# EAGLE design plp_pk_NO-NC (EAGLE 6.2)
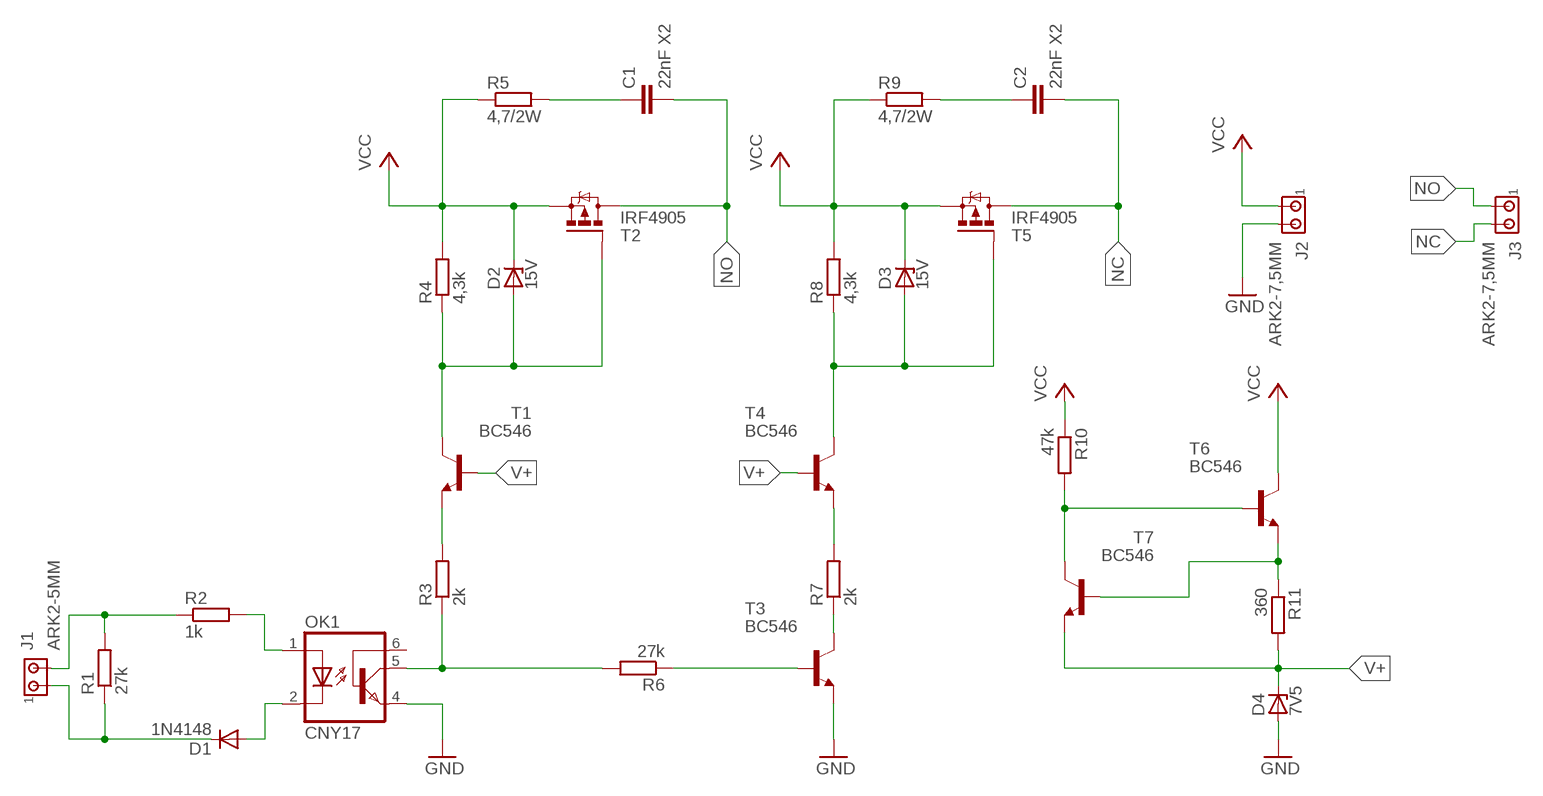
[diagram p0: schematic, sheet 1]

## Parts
C1  22nF X2  C-EU102-054X133  [C102-054X133]
C2  22nF X2  C-EU102-054X133  [C102-054X133]
D1  1N4148  1N4148DO35-7  [DO35-7]
D2  15V  ZENER-DIODEDO34-7  [DO34Z7]
D3  15V  ZENER-DIODEDO34-7  [DO34Z7]
D4  7V5  ZENER-DIODEDO34-7  [DO34Z7]
J1  ARK2-5MM  [2PIN-5MM]
J2  ARK2-7,5MM  [2PIN-7,5MM]
J3  ARK2-7,5MM  [2PIN-7,5MM]
OK1  CNY17  [DIL06]
R1  27k  R-EU_0207/7  [0207/7]
R2  1k  R-EU_0207/7  [0207/7]
R3  2k  R-EU_0207/7  [0207/7]
R4  4,3k  R-EU_0207/7  [0207/7]
R5  4,7/2W  R-EU_0613/5V  [P0613V]
R6  27k  R-EU_0207/7  [0207/7]
R7  2k  R-EU_0207/7  [0207/7]
R8  4,3k  R-EU_0207/7  [0207/7]
R9  4,7/2W  R-EU_0613/5V  [P0613V]
R10  47k  R-EU_0207/7  [0207/7]
R11  360  R-EU_0207/7  [0207/7]
T1  BC546  MPSA42-NPN-TO92-CBE  [TO92-CBE]
T2  IRF4905  IRF9530  [TO220BV]
T3  BC546  MPSA42-NPN-TO92-CBE  [TO92-CBE]
T4  BC546  MPSA42-NPN-TO92-CBE  [TO92-CBE]
T5  IRF4905  IRF9530  [TO220BV]
T6  BC546  MPSA42-NPN-TO92-CBE  [TO92-CBE]
T7  BC546  MPSA42-NPN-TO92-CBE  [TO92-CBE]

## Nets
GND: D4.A J2.P2 OK1.4(EMI) T3.E
N$1: OK1.1(A) R2.2
N$2: D1.A OK1.2(C)
N$3: D1.C J1.P$1 R1.1
N$4: J1.P$2 R1.2 R2.1
N$5: OK1.5(COL) R3.1 R6.2
N$6: R3.2 T1.E
N$7: D2.A R4.1 T1.C T2.G
N$8: C1.1 R5.2
N$9: R11.1 T6.E T7.B
N$10: R6.1 T3.B
N$11: R7.1 T3.C
N$12: D3.A R8.1 T4.C T5.G
N$13: R7.2 T4.E
N$14: C2.1 R9.2
N$18: R10.2 T6.B T7.C
NC: C2.2 J3.P2 T5.D
NO: C1.2 J3.P1 T2.D
V+: D4.C R11.2 T1.B T4.B T7.E
VCC: D2.C D3.C J2.P1 R4.2 R5.1 R8.2 R9.1 R10.1 T2.S T5.S T6.C
Unconnected: OK1.6(BAS)

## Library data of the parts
C1 C2 = rcl:C-EU: CAPACITOR, European symbol
D1 = diode:1N4148: DIODE
D2-D4 = diode:ZENER-DIODE: Z-Diode
J1-J3 = zlacza_futrzak:ARK2: ARK 2
OK1 = optocoupler:CNY17: SIEMENS OPTO COUPLER; MPN: CNY17-1; OC_FARNELL: 1045399; OC_NEWARK: 05M4044
R1-R11 = rcl:R-EU_: RESISTOR, European symbol
T1 T3 T4 T6 T7 = transistor:*-NPN-: NPN Transistror BF959 corrected 2008.03.06
T2 T5 = transistor-power:IRF9530: P-CHANNEL HEXFET POWER-MOS-FET Source: http://www.irf.com/product-info/datasheets/data/irf9530.pdf

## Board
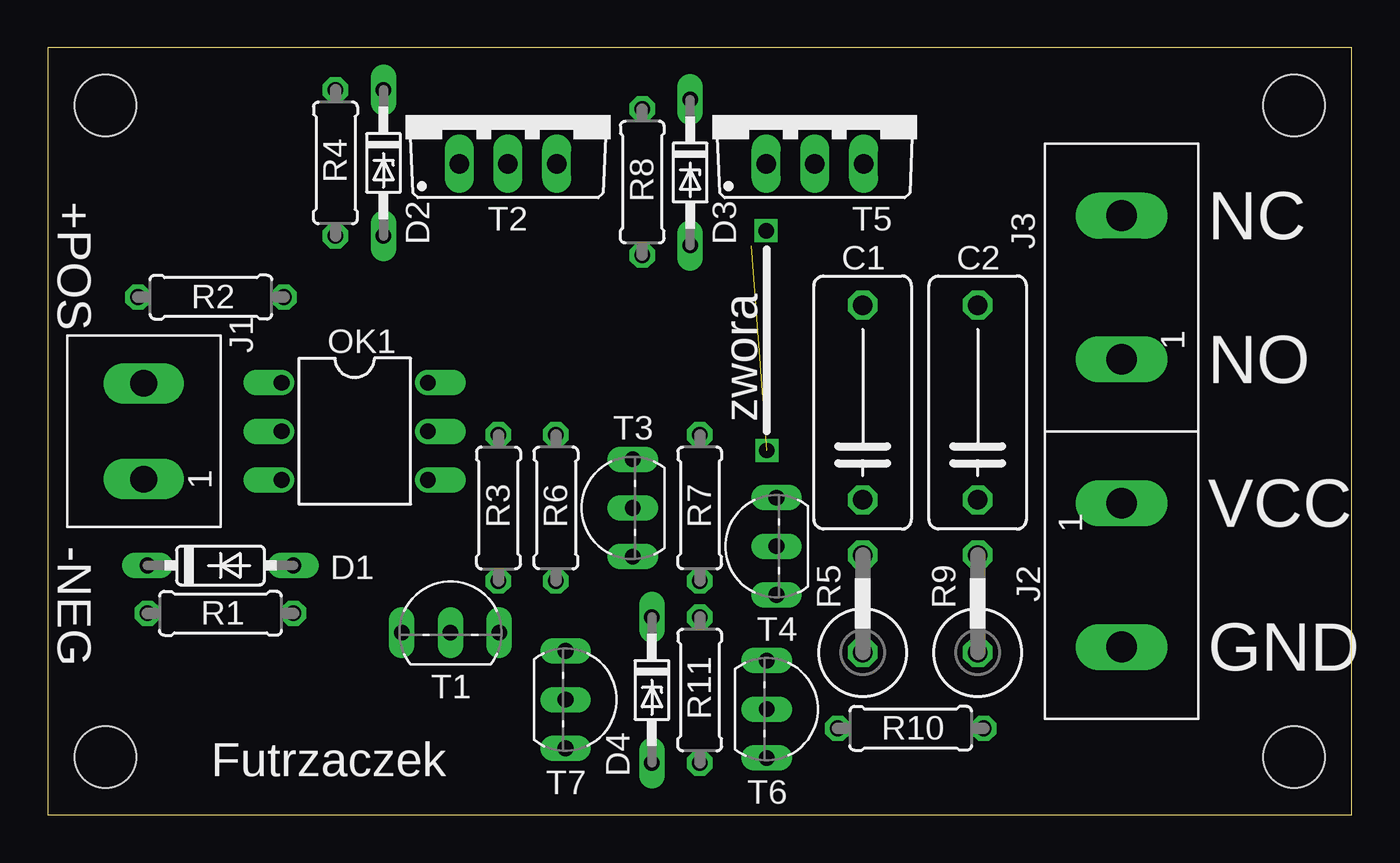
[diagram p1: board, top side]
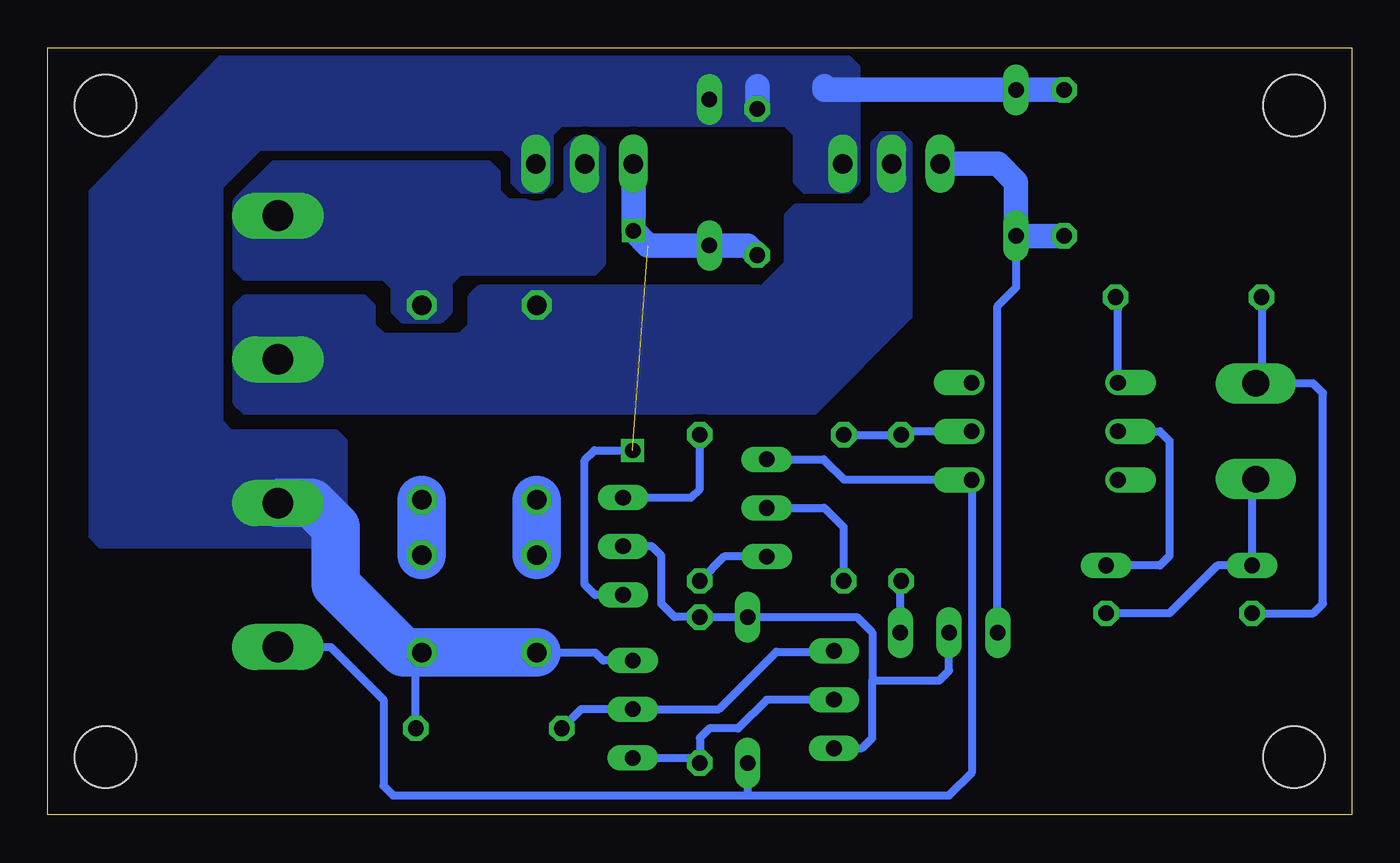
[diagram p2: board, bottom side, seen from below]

Size 68 x 40 mm. Coordinates in mm from the lower left corner, seen from the top.
Outline: 0,0 68,0 68,40 0,40 0,0
Copper layers (1*16): Top 0.035mm / dielectric 1.5mm / Bottom 0.035mm
Design rules: minimum track width 10mil, minimum drill 24mil, track to track 8mil, track to pad 8mil, pad to pad 8mil, via to via 8mil, smd to smd 8mil, copper to edge 10mil, drill to drill 8mil, minimum pad ring 10mil, minimum via ring 8mil, stop-mask expansion 4mil, vias tented up to drill 0mil, thermal gap 10mil
Holes 3.2 mm at 3,3 3,37 65,37 65,3

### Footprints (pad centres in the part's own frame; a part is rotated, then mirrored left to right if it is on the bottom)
C102-054X133 = drill 1.016 octagon: 1 -5.08,0; 2 5.08,0
DO35-7 = drill 0.813 long: A 3.81,0; C -3.81,0
DO34Z7 = drill 0.813 long: A 3.81,0; C -3.81,0
2PIN-5MM = drill 1.4 long: P$1 -2.5,0; P$2 2.5,0
2PIN-7,5MM = drill 1.6 long: P1 -3.75,0; P2 3.75,0
DIL06 = drill 0.813 offset: 1 -2.54,-3.81; 2 0,-3.81; 3 2.54,-3.81; 4 2.54,3.81; 5 0,3.81; 6 -2.54,3.81
0207/7 = drill 0.813 octagon: 1 -3.81,0; 2 3.81,0
P0613V = drill 1.016 octagon: 1 -2.54,0; 2 2.54,0
TO92-CBE = drill 0.813 long: B 0,0; C -2.54,0; E 2.54,0
TO220BV = drill 1.016 long: D 0,-2.54; G -2.54,-2.54; S 2.54,-2.54

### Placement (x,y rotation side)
C1  42.5,21.5 90 top
C2  48.5,21.5 90 top
D1  9,13 0 top
D2  17.5,34 270 top
D3  33.5,33.5 270 top
D4  31.5,6.5 270 top
J1  5,20 90 top
J2  56,12.5 270 top
J3  56,27.5 90 top
OK1  16,20 270 top
R1  9,10.5 180 top
R2  8.5,27 0 top
R3  23.5,16 270 top
R4  15,34 90 top
R5  42.5,11 90 top
R6  26.5,16 90 top
R7  34,16 90 top
R8  31,33 90 top
R9  48.5,11 90 top
R10  45,4.5 180 top
R11  34,6.5 90 top
T1  21,9.5 0 top
T2  24,36.5 0 top
T3  30.5,16 90 top
T4  38,14 90 top
T5  40,36.5 0 top
T6  37.5,5.5 270 top
T7  27,6 270 top

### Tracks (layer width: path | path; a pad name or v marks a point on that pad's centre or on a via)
GND
  Bottom 0.406: J2.P2 53.25,8.75 50.5,6 50.5,1.5 50,1 31.5,1 | 31.5,1 21,1 19.81,2.19 OK1.4 26.46,17.46 27.54,18.54 T3.E | D4.A 31.5,1
N$1
  Bottom 0.406: OK1.1 12.19,26.38 R2.2
N$2
  Bottom 0.406: OK1.2 10,20 9.5,19.5 9.5,13.5 10,13 D1.A
N$3
  Bottom 0.406: J1.P$1 5.19,17.31 D1.C 7,13 9.5,10.5 R1.1
N$4
  Bottom 0.406: R1.2 2,10.5 1.5,11 1.5,22 2,22.5 4.5,22.5 | 4.5,22.5 J1.P$2 | R2.1 4.69,22.69 4.5,22.5
N$5
  Bottom 0.406: R6.2 R3.1 23.31,20 OK1.5
N$6
  Bottom 0.406: T1.E 23.54,12.15 R3.2
N$7
  Bottom 0.406: D2.A 17.5,27.5 18.5,26.5 18.5,9.54 T1.C
  Bottom 1.27: T2.G 18.46,33.96 17.5,33 D2.A R4.1
N$8
  Bottom 2.54: R5.2 C1.1
N$9
  Bottom 0.406: T6.E 34.27,2.96 R11.1 34,4 33.5,4.5 32,4.5 30.5,6 T7.B
N$10
  Bottom 0.406: T3.B 27.5,16 26.5,15 R6.1
N$11
  Bottom 0.406: T3.C 32.73,13.46 R7.1
N$12  (via drill 0.8)  (1 unrouted)
  Bottom 0.406: T4.C 39.46,11.46 40,12 40,18.5 39.5,19 v37.5,19
  Bottom 1.27: T5.G v37.46,30.46 36.69,29.69 D3.A 31.5,29.69 R8.1
N$13
  Bottom 0.406: T4.E 34.46,16.54 34,17 R7.2
N$14
  Bottom 2.54: R9.2 C2.1
N$18
  Bottom 0.406: R10.2 40.19,5.5 T6.B 33,5.5 30,8.5 27.04,8.5 T7.C
NC
  pour Bottom (isolate 0.406, no thermals): 39,34.75 39.5,35.25 40.5,35.25 41,34.75 41,32.5 41.5,32 44,32 44.5,32.5 44.5,33.5 45,34 56.25,34 58.25,32 58.25,28.5 57.75,28 50.5,28 50,27.5 50,26.25 49.5,25.75 47.5,25.75 47,26.25 47,27.75 46.5,28.25 39.5,28.25 39,28.75
NO
  pour Bottom (isolate 0.406, no thermals): 23.5,35.5 24.5,35.5 25,35 25,32.25 25.5,31.75 29,31.75 29.5,31.25 29.5,28.75 30.75,27.5 45.5,27.5 46,27 46,25.5 46.5,25 50.5,25 51,25.5 51,26.5 51.5,27 57.75,27 58.25,26.5 58.25,21.5 57.75,21 28,21 23,26 23,35
V+
  Bottom 0.406: T7.E 25.54,3.46 25,4 25,7 | 25,7 25,9.5 25.81,10.31 D4.C R11.2 35.31,10.31 36,11 36,13.5 36.5,14 T4.B | 25,7 21.5,7 21,7.5 T1.B
VCC
  Bottom 0.406: T6.C 39.04,8.04 39.46,8.46 R5.1 | R10.1 48.81,8.15 R9.1
  Bottom 1.27: 27.5,38 27.5,37.81 D2.C R4.2 | R8.2 31,38
  Bottom 2.54: R5.1 R9.1 49.46,8.46 53,12 53,15 54.25,16.25 J2.P1
  pour Bottom (isolate 0.406, no thermals): 25.75,39 25.75,33 26.25,32.5 28.5,32.5 29,33 29,35.5 29.5,36 41.25,36 41.75,35.5 41.75,33 42.25,32.5 43.25,32.5 43.75,33 43.75,34.25 44.25,34.75 57,34.75 59,32.75 59,20.5 58.5,20 53,20 52.5,19.5 52.5,14.5 53,14 65.25,14 65.75,14.5 65.75,32.5 59,39.5 26.25,39.5

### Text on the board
tPlace: +POS | NC | NO | zwora | VCC | -NEG | GND | Futrzaczek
